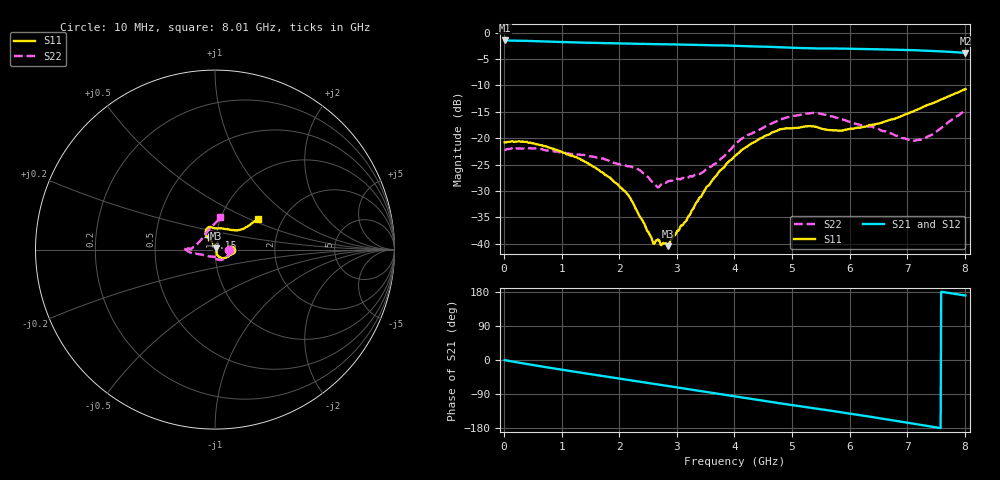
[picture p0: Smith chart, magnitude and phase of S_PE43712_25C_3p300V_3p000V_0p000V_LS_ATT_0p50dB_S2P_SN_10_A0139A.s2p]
! DEVICE ID: PE43712
! File Path: z:\PE43713\PE43713_CHAR_NOM_04292014\AMB\3p300\LS_ATT_0p50dB\PE43713_AMB_3p300V_3p000V_0p000V_LS_ATT_0p50dB_S2P_SN_10_A0139A.s2p
! Serial: 10
! Lot: A0139A
! Temp: 25C
! VDD: 3.300
! VSS: 0.000
! Control_Hi: 3.000
! Control_Lo: 0.000
! Attenuation Step: 0.50dB
! Port 1: RF1
! Port 2: RF2
! ThroughPath:1-2
! IDD: 0.0001467518
! ISS: -3.24e-008
#  Hz  S  RI  R  50
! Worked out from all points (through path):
!   801 points, 10 MHz to 8.01 GHz, reference 50 ohm
!   highest |S21| = -1.48 dB at 10 MHz (marker M1); lowest = -3.8 dB at 8.01 GHz (marker M2)
!   group delay of S21, straight-line fit = 65 ps
!   lowest |S11| = -40.5 dB at 2.84 GHz (marker M3), VSWR 1.02, Z = 50.7 + j0.643 ohm
!   |S11| at or under -10 dB: start of sweep to end of sweep
!   |S22| runs from -29.3 to -14.8 dB; largest |S21 - S12| = 0.0028
!   S11 on the Smith chart (normalised r, x): 10 MHz: 1.20, -0.00; 4.15 GHz: 0.91, +0.12; 8.01 GHz: 1.50, +0.55
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1e7  0.0914 -0.000616  0.8435 -0.00449  0.8434 -0.00417  0.0777 -0.00086
3.6e8  0.0895 -0.0232  0.8234 -0.1388  0.8256 -0.1383  0.0758 -0.0224
6.9e8  0.0757 -0.0371  0.7854 -0.2551  0.7849 -0.255  0.0677 -0.0375
1.35e9  0.04 -0.0473  0.6687 -0.4483  0.6682 -0.4481  0.0397 -0.0569
1.82e9  0.0205 -0.0376  0.5636 -0.5591  0.5633 -0.5588  0.0224 -0.0569
2.11e9  0.0107 -0.0292  0.4904 -0.6173  0.4902 -0.6169  0.0103 -0.0543
2.35e9  0.00815 -0.0165  0.4248 -0.6584  0.4249 -0.6581  0.00758 -0.0494
2.58e9  0.00983 -0.00386  0.3593 -0.6892  0.3595 -0.6893  0.00494 -0.038
2.68e9  0.0108 0.00179  0.332 -0.7016  0.3323 -0.7012  0.00778 -0.0334
2.84e9  0.00707 0.00634  0.2844 -0.721  0.2847 -0.721  0.00126 -0.0389
3.14e9  -0.0016 0.016  0.192 -0.7458  0.1921 -0.7455  -0.0138 -0.0389
3.43e9  -0.0076 0.0274  0.1011 -0.7562  0.1014 -0.7565  -0.0277 -0.0379
3.74e9  -0.0174 0.0456  0.00518 -0.7582  0.00601 -0.758  -0.0516 -0.034
4.01e9  -0.0318 0.0597  -0.0794 -0.7471  -0.0788 -0.7468  -0.0829 -0.0272
4.15e9  -0.0402 0.0676  -0.1218 -0.7366  -0.1211 -0.7364  -0.0979 -0.0243
4.78e9  -0.0504 0.1099  -0.2959 -0.6643  -0.2953 -0.6647  -0.1489 -0.0103
5.35e9  -0.0302 0.1261  -0.4247 -0.57  -0.4244 -0.5693  -0.1735 0.00683
5.85e9  0.0117 0.1172  -0.5245 -0.4732  -0.5233 -0.4735  -0.1518 0.00498
6.68e9  0.1001 0.1087  -0.6384 -0.2641  -0.6382 -0.2634  -0.1105 0.0198
7.05e9  0.1366 0.1097  -0.6654 -0.1585  -0.6648 -0.1584  -0.0807 0.051
7.26e9  0.1585 0.1155  -0.6703 -0.0965  -0.6695 -0.0962  -0.0595 0.0772
8.01e9  0.2381 0.1679  -0.6342 0.1095  -0.632 0.1083  0.0292 0.1796
